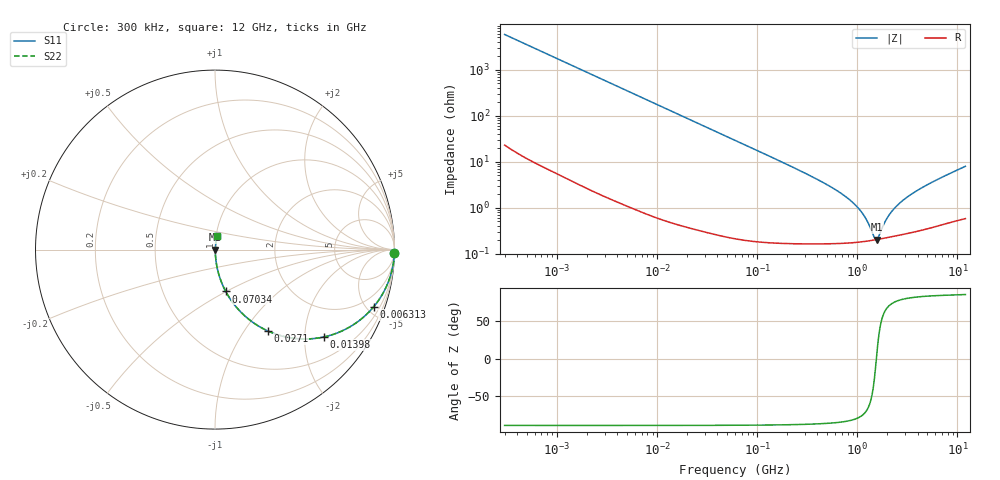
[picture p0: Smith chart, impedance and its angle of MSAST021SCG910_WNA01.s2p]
! MSAST021SCG910_WNA01  S-PARAMETER MODEL  ( Standard Model )
! Model Generated by TAIYO YUDEN Corporation (http://www.ty-top.com)
! Version 1.0
! TAIYO YUDEN Control No. 241126
! Copyright(c) 2024 TAIYO YUDEN CO.,LTD. All Rights Reserved.
! Product Description (link to TY-COMPAS)
! https://ds.yuden.co.jp/TYCOMPAS/or/detail?pn=MSAST021SCG910GWNA01&u=M
! Products Name : Multilayer Ceramic Capacitors
! Characteristics :
!  Capacitance : 91 [pF] , Rated Voltage : 25 [V] , TCC : CG / C0G
!  Case Size : 0.25 x 0.125 / 0.0098 x 0.0049 [mm/inch] , Thickness : 0.125 / 0.0049 [mm/inch]
!  (Conditions: Temperature = 25 [degC] , DC Bias Voltage = 0 [V])
! External Node Assignments :
!  1  o---| |---o  2
! GND o---------o GND
! Frequency Range : 0.3MHz  -  12000MHz  [ 401 STEP ]
# MHZ S RI R 50
! Freq[MHz].  S11 Real  S11 Imag  S21 Real  S21 Imag  S12 Real  S12 Imag  S22 Real  S22 Imag
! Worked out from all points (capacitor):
!   401 points, 300 kHz to 12 GHz, reference 50 ohm
!   read as one part in series: C = 91.8 pF near 316.3 kHz
!   lowest |Z| = 203 mohm at 1.561 GHz (marker M1)
!   series resonance near 1.55 GHz, so ESL is about 110 pH
!   S11 on the Smith chart (normalised r, x): 300 kHz: open; 6.313 MHz: 1.02, -5.52; 13.98 MHz: 1.01, -2.50; 27.1 MHz: 1.01, -1.29; 70.34 MHz: 1.00, -0.50; 12 GHz: 1.01, +0.16
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0.3  0.9996 -0.0173  0.000368 0.0173  0.000368 0.0173  0.9996 -0.0173
1.769972  0.9894 -0.1007  0.0106 0.1007  0.0106 0.1007  0.9894 -0.1007
3.716298  0.9558 -0.204  0.0442 0.204  0.0442 0.204  0.9558 -0.204
6.312676  0.8831 -0.3197  0.1169 0.3197  0.1169 0.3197  0.8831 -0.3197
10.44266  0.7352 -0.4395  0.2648 0.4395  0.2648 0.4395  0.7352 -0.4395
13.97552  0.6085 -0.4862  0.3915 0.4862  0.3915 0.4862  0.6085 -0.4862
27.10171  0.2941 -0.4532  0.7059 0.4532  0.7059 0.4532  0.2941 -0.4532
60  0.0797 -0.2672  0.9203 0.2672  0.9203 0.2672  0.0797 -0.2672
70.33673  0.0596 -0.2328  0.9404 0.2328  0.9404 0.2328  0.0596 -0.2328
147.6816  0.0152 -0.1154  0.9848 0.1154  0.9848 0.1154  0.0152 -0.1154
353.9943  0.0038 -0.0466  0.9962 0.0466  0.9962 0.0466  0.0038 -0.0466
634.0297  0.00218 -0.0228  0.9978 0.0228  0.9978 0.0228  0.00218 -0.0228
918.7169  0.00188 -0.0122  0.9981 0.0122  0.9981 0.0122  0.00188 -0.0122
1166.079  0.00187 -0.00643  0.9981 0.00643  0.9981 0.00643  0.00187 -0.00643
1480.043  0.00198 -0.00102  0.998 0.00102  0.998 0.00102  0.00198 -0.00102
1560.575  0.00202 0.000156  0.998 -0.000156  0.998 -0.000156  0.00202 0.000156
1645.489  0.00206 0.00133  0.9979 -0.00133  0.9979 -0.00133  0.00206 0.00133
1878.541  0.00219 0.00426  0.9978 -0.00426  0.9978 -0.00426  0.00219 0.00426
2088.533  0.00232 0.00664  0.9977 -0.00664  0.9977 -0.00664  0.00232 0.00664
2650.866  0.00267 0.0122  0.9973 -0.0122  0.9973 -0.0122  0.00267 0.0122
3740.715  0.00342 0.0215  0.9966 -0.0215  0.9966 -0.0215  0.00342 0.0215
12000  0.0118 0.0774  0.9882 -0.0774  0.9882 -0.0774  0.0118 0.0774
